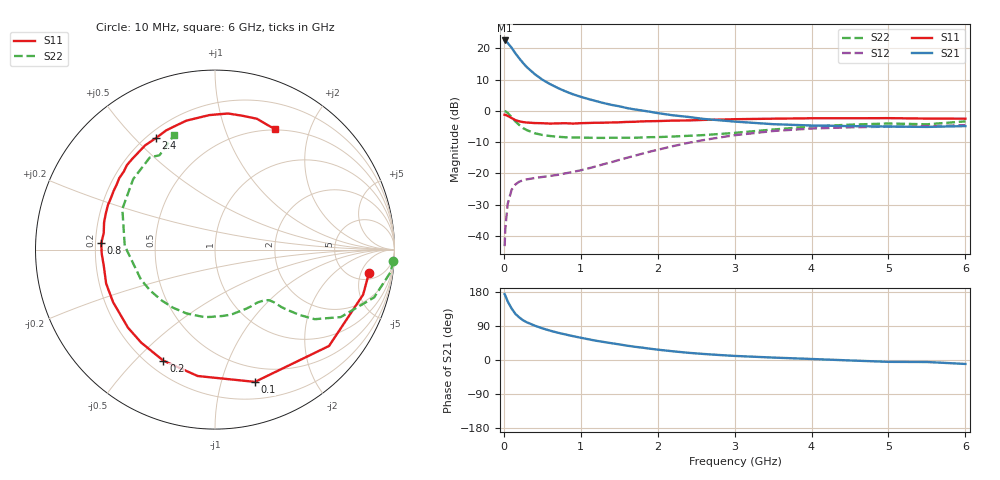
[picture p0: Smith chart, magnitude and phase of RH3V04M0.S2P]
! SIEMENS Small Signal Semiconductors
! BFR106
! Si NPN RF Bipolar Junction Transistor in SOT23
! VCE = 3 V  IC = 4 mA
! Common Emitter S-Parameters:  August  1996
# GHz  S  MA  R  50
!  f  S11  S21  S12  S22
! GHz  MAG  ANG  MAG  ANG  MAG  ANG  MAG  ANG
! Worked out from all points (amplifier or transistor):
!   36 points, 10 MHz to 6 GHz, reference 50 ohm
!   highest |S21| = 22.5 dB at 10 MHz (marker M1)
!   |S21| within 3 dB of that: start of sweep to 119.6 MHz
!   unconditionally stable (mu >= 1): 658.8 MHz to 2.043 GHz; 4.343 GHz to end of sweep
!   at 250 MHz: K = 0.45, MSG = 18.7 dB, |S12| = -22.2 dB
!   at 1.4 GHz: K = 1.19, MAG = 6.5 dB, |S12| = -16.4 dB
!   at 6 GHz: K = 1.02, MAG = -1.1 dB, |S12| = -4.6 dB
!   S11 on the Smith chart (normalised r, x): 10 MHz: 6.76, -7.02; 100 MHz: 0.36, -1.28; 200 MHz: 0.26, -0.61; 800 MHz: 0.22, +0.03; 2.4 GHz: 0.23, +0.58; 6 GHz: 0.49, +1.51
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0.01  0.8678 -8.5  13.32 174.0  0.0069 86.5  0.9943 -3.6
0.02  0.8626 -16.9  13.13 169.7  0.0136 80.1  0.9872 -7.2
0.05  0.8318 -40.2  12.15 154.7  0.0326 69.1  0.9258 -16.7
0.1  0.7698 -73.2  10.24 136.2  0.0546 54.9  0.7953 -28.2
0.15  0.7109 -97.8  8.295 121.8  0.0668 44.9  0.6777 -34.9
0.2  0.6825 -114.9  6.91 112.5  0.0739 39.8  0.5955 -37.7
0.25  0.6616 -128.4  5.81 104.8  0.0779 36.3  0.5309 -39.6
0.3  0.6514 -138.1  4.981 99.4  0.0806 34.8  0.4921 -40.8
0.4  0.6389 -152.7  3.877 90.8  0.0845 34.2  0.4399 -41.8
0.5  0.6353 -162.7  3.155 83.6  0.0879 35.7  0.4123 -43.1
0.6  0.6263 -171.4  2.679 77.5  0.0914 38.2  0.3968 -45.3
0.8  0.6347 176.8  2.051 67.4  0.1004 44.0  0.3786 -51.0
1.1  0.6408 161.7  1.545 54.7  0.1207 53.0  0.3725 -61.9
1.3  0.6472 153.6  1.33 47.5  0.141 57.2  0.3701 -70.0
1.6  0.6658 143.2  1.109 37.9  0.1778 60.6  0.3723 -83.7
2.2  0.6991 123.9  0.849 22.9  0.2735 58.4  0.3893 -114.1
2.4  0.7032 117.9  0.8 19.0  0.3086 55.7  0.3996 -125.9
3.5  0.7501 92.4  0.613 6.4  0.4766 34.8  0.5033 177.6
4.5  0.7613 78.0  0.571 -1.2  0.5458 15.2  0.6019 139.2
5  0.7654 72.2  0.562 -4.9  0.5594 7.4  0.6287 125.3
5.5  0.7532 67.0  0.554 -5.3  0.5672 3.6  0.61 120.4
6  0.7496 63.3  0.571 -10.4  0.5918 -4.1  0.6792 109.5
